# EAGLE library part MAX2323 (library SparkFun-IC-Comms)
RS232 Transceiver This part covers 232 drivers that are compatible with the MAX3232. Sipex SP3232EB Datasheet SparkFun Products SOIC component (COM-00589 / IC-08171) Retired DIP component (COM-00316 / IC-08446) SparkFun Transceiver Breakout - MAX3232 (BOB-11189) SparkFun XBee Explorer Serial (WRL-13225)
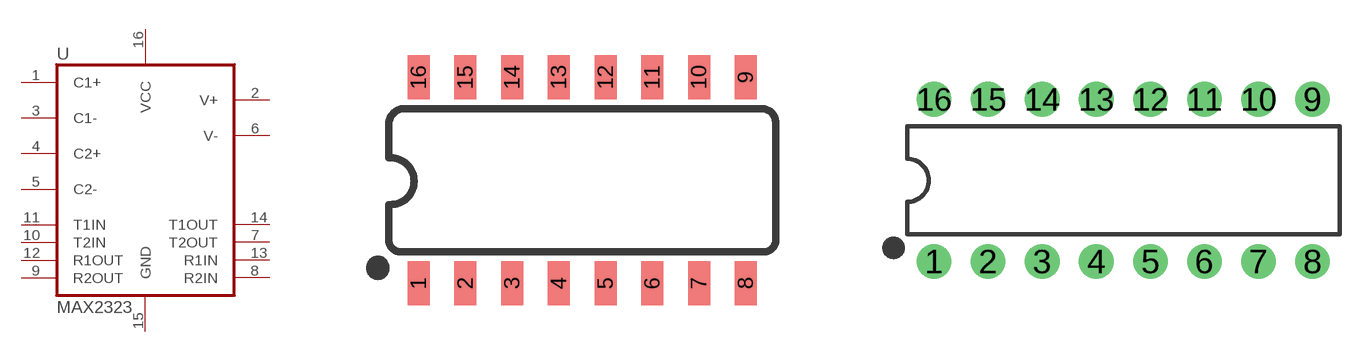
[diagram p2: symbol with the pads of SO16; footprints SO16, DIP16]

Designator prefix U

## MAX2323SOIC16 (PROD_ID: IC-08171; VALUE: MAX3232)  [SO16]
1  C1+
2  V+
3  C1-
4  C2+
5  C2-
6  V-
7  T2OUT  out
8  R2IN  in
9  R2OUT  out
10  T2IN  in
11  T1IN  in
12  R1OUT  out
13  R1IN  in
14  T1OUT  out
15  GND
16  VCC

## MAX2323PTH (PROD_ID: IC-08446; VALUE: MAX3232)  [DIP16]
Pads as for SO16

## MAX2323TSSOP (PROD_ID: NA-XXXXX; VALUE: MAX3232)  [TSSOP16]
Pads as for SO16

## Footprint SO16 (pad centres in mm)
SOIC-16 Specifications: Pin count: 16 Width:0.15" Example device(s): HEX_CONVERTER
smd 0.6 x 1.2: 1 -4.445,-2.8; 2 -3.175,-2.8; 3 -1.905,-2.8; 4 -0.635,-2.8; 5 0.635,-2.8; 6 1.905,-2.8; 7 3.175,-2.8; 8 4.445,-2.8; 9 4.445,2.8; 10 3.175,2.8; 11 1.905,2.8; 12 0.635,2.8; 13 -0.635,2.8; 14 -1.905,2.8; 15 -3.175,2.8; 16 -4.445,2.8

## Footprint DIP16 (pad centres in mm)
Dual In Line Package - 16 Specifications: Pin count:16 Example device(s): MAX2323
drill 0.813 pad 1.626: 1 -8.89,-3.81; 2 -6.35,-3.81; 3 -3.81,-3.81; 4 -1.27,-3.81; 5 1.27,-3.81; 6 3.81,-3.81; 7 6.35,-3.81; 8 8.89,-3.81; 9 8.89,3.81; 10 6.35,3.81; 11 3.81,3.81; 12 1.27,3.81; 13 -1.27,3.81; 14 -3.81,3.81; 15 -6.35,3.81; 16 -8.89,3.81

## Footprint TSSOP16 (pad centres in mm)
TSOP16 thin small outline package
smd 0.4 x 1.6: 1 -2.225,-2.85; 2 -1.575,-2.85; 3 -0.925,-2.85; 4 -0.275,-2.85; 5 0.375,-2.85; 6 1.025,-2.85; 7 1.675,-2.85; 8 2.325,-2.85; 9 2.325,3.05; 10 1.675,3.05; 11 1.025,3.05; 12 0.375,3.05; 13 -0.275,3.05; 14 -0.925,3.05; 15 -1.575,3.05; 16 -2.225,3.05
